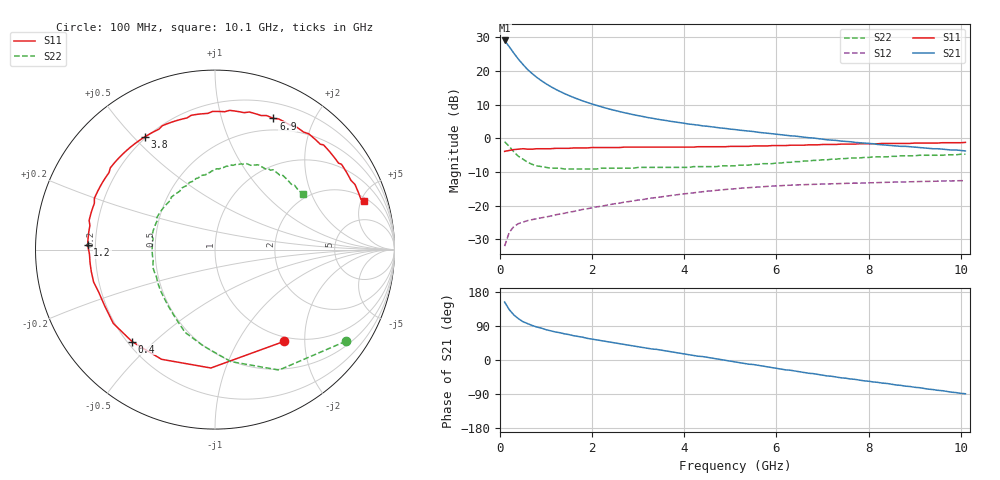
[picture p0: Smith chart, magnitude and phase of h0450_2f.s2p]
!HBFP-0450
!S and NOISE PARAMETERS at Vce=2V  Ic=20mA.  LAST UPDATED  09-04-98
# GHZ S MA R  50
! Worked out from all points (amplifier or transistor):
!   101 points, 100 MHz to 10.1 GHz, reference 50 ohm
!   highest |S21| = 29.1 dB at 100 MHz (marker M1)
!   |S21| within 3 dB of that: start of sweep to 260.1 MHz
!   unconditionally stable (mu >= 1): 2.371 GHz to end of sweep
!   at 1.7 GHz: K = 0.88, MSG = 16.5 dB, |S12| = -21.4 dB
!   at 5.1 GHz: K = 1.10, MAG = 6.9 dB, |S12| = -15.0 dB
!   at 10.1 GHz: K = 1.05, MAG = 3.0 dB, |S12| = -12.6 dB
!   lowest NFmin = 1.30 dB at 1.8 GHz
!   S11 on the Smith chart (normalised r, x): 100 MHz: 0.92, -1.60; 400 MHz: 0.22, -0.43; 1.2 GHz: 0.17, +0.02; 3.8 GHz: 0.19, +0.54; 6.9 GHz: 0.36, +1.48; 10.1 GHz: 2.38, +5.27
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0.1  0.64 -53.0  28.41 153.0  0.025 67.0  0.89 -35.0
0.2  0.66 -92.0  22.98 133.0  0.04 51.0  0.76 -62.0
0.3  0.68 -116.0  18.41 119.0  0.049 42.0  0.63 -82.0
0.4  0.69 -132.0  14.96 109.0  0.054 37.0  0.54 -97.0
0.5  0.7 -144.0  12.45 101.0  0.057 33.0  0.49 -110.0
0.6  0.69 -153.0  10.5 96.0  0.06 32.0  0.44 -120.0
0.7  0.69 -160.0  9.11 91.0  0.062 31.0  0.41 -129.0
0.8  0.7 -165.0  8.02 87.0  0.064 30.0  0.39 -137.0
0.9  0.7 -170.0  7.16 84.0  0.066 30.0  0.38 -143.0
1  0.7 -174.0  6.45 80.0  0.068 30.0  0.37 -149.0
1.2  0.71 178.0  5.38 74.0  0.073 30.0  0.36 -160.0
1.4  0.71 172.0  4.61 69.0  0.077 30.0  0.35 -170.0
1.8  0.72 162.0  3.58 60.0  0.088 29.0  0.35 179.0
2.1  0.73 155.0  3.08 53.0  0.096 28.0  0.35 170.0
2.5  0.73 147.0  2.59 45.0  0.107 26.0  0.36 161.0
3.5  0.74 127.0  1.88 26.0  0.135 18.0  0.37 143.0
3.8  0.74 122.0  1.75 20.0  0.144 15.0  0.37 137.0
5.1  0.76 98.0  1.35 -5.0  0.178 -1.0  0.39 113.0
6.8  0.8 68.0  1.01 -36.0  0.207 -24.0  0.47 82.0
6.9  0.8 66.0  0.99 -38.0  0.208 -26.0  0.47 81.0
8.5  0.84 41.0  0.78 -64.0  0.223 -47.0  0.54 57.0
10.1  0.87 18.0  0.65 -89.0  0.234 -69.0  0.58 32.0
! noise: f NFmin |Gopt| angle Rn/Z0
1.8  1.3  0.49  -166  0.06
2  1.34  0.5  -164  0.06
2.5  1.47  0.54  -152  0.08
3.5  1.72  0.61  -133  0.18
4  1.87  0.64  -121  0.29
5  2.12  0.68  -102  0.57
5.5  2.26  0.71  -91  0.82
7  2.63  0.76  -64  1.8
8  2.89  0.8  -47  2.71
10  3.4  0.82  -18  4.58
